|Texas Instruments Incorporated
|tmux7348f,  ±60-V Fault-Protected, 8:1 with configurable fault thresholds
[IBIS Ver]   4.1
[File name]   tmux7348f.ibs
[Date]   01/21/22
[File Rev]   1.0
[Source]
| Texas Instruments Incorporated.
| ASC-INT-MPD
| 12500 TI Blvd
| Dallas, TX - 75243
[Notes]   Revision History:
| Rev 1.0: 01/21/22
| - Initial version of the model
| - Model generated from simulations in SPECTRE
| - C_comp although listed in numerical order of value are
|   obtained from varying PVT conditions. For PVT conditions for
|   each specific value refer the buffer description under
|   respective [Model]. IBIS model user is responsible for using
|   appropriate C_comp to simulate for Signal Integrity.
[Disclaimer]
| This model is designed as an aid for customers of Texas Instruments.
| TI and its licensors and suppliers make no warranties, either expressed
| or implied, with respect to this  model, including the warranties of
| merchantability or fitness for a particular purpose. The model is
| provided solely on an "as is" basis. The entire risk as to its quality
| and performance is with the customer.
| This model is subject to change without notice. Texas Instruments
| Incorporated is not responsible for updating this model.
[Copyright]
(C) Copyright 2022 Texas Instruments Incorporated.All rights reserved.
|  Component TMUX7348FPW 20-pin - PW package
|  Part # TMUX7348FPW
[Component]   TMUX7348FPW
[Manufacturer]  TI
[Package]
|   typ   min   max
R_pkg   0.0668   NA   NA
L_pkg   2.1992nH   NA   NA
C_pkg   0.2884pF   NA   NA
[Pin]   signal_name   model_name
   1   A0   inbuf
   2   EN   inbuf
   3   VSS   POWER
   4   S1   sterm
   5   S2   sterm
   6   S3   sterm
   7   S4   sterm
   8   D   dterm
   9   VFN   nfault
   10   SF   ofault
   11   FF   ofault
   12   VFP   pfault
   13   S8   sterm
   14   S7   sterm
   15   S6   sterm
   16   S5   sterm
   17   VDD   POWER
   18   GND   GND
   19   A2   inbuf
   20   A1   inbuf
[Series Switch Groups]
On 1 /
On 2 /
On 3 /
On 4 /
On 5 /
On 6 /
On 7 /
On 8 /
Off 1 2 3 4 5 6 7 8 /
[Series Pin Mapping]  pin_2 model_name function_table_group
   4   8   switch_dual_20   1
   5   8   switch_dual_20   2
   6   8   switch_dual_20   3
   7   8   switch_dual_20   4
  16   8   switch_dual_20   5
  15   8   switch_dual_20   6
  14   8   switch_dual_20   7
  13   8   switch_dual_20   8
|   4   8   switch_36   1
|   5   8   switch_36   2
|   6   8   switch_36   3
|   7   8   switch_36   4
|  16   8   switch_36   5
|  15   8   switch_36   6
|  14   8   switch_36   7
|  13   8   switch_36   8
|   4   8   switch_dual_15   1
|   5   8   switch_dual_15   2
|   6   8   switch_dual_15   3
|   7   8   switch_dual_15   4
|  16   8   switch_dual_15   5
|  15   8   switch_dual_15   6
|  14   8   switch_dual_15   7
|  13   8   switch_dual_15   8
|   4   8   switch_12   1
|   5   8   switch_12   2
|   6   8   switch_12   3
|   7   8   switch_12   4
|  16   8   switch_12   5
|  15   8   switch_12   6
|  14   8   switch_12   7
|  13   8   switch_12   8
|  Component TMUX7348FRRP 20-pin - RRP package
|  Part # TMUX7348FRRP
[Component]   TMUX7348FRRP
[Manufacturer]  TI
[Package]
|   typ   min   max
R_pkg   0.067   NA   NA
L_pkg   0.937nH   NA   NA
C_pkg   0.144pF   NA   NA
[Pin]   signal_name   model_name
   1   VSS   POWER
   2   S1   sterm
   3   S2   sterm
   4   S3   sterm
   5   S4   sterm
   6   D   dterm
   7   VFN   nfault
   8   SF   ofault
   9   FF   ofault
   10   VFP   pfault
   11   S8   sterm
   12   S7   sterm
   13   S6   sterm
   14   S5   sterm
   15   VDD   POWER
   16   GND   GND
   17   A2   inbuf
   18   A1   inbuf
   19   A0   inbuf
   20   EN   inbuf
[Series Switch Groups]
On 1 /
On 2 /
On 3 /
On 4 /
On 5 /
On 6 /
On 7 /
On 8 /
Off 1 2 3 4 5 6 7 8 /
[Series Pin Mapping]  pin_2 model_name function_table_group
   2   6   switch_dual_20   1
   3   6   switch_dual_20   2
   4   6   switch_dual_20   3
   5   6   switch_dual_20   4
  14   6   switch_dual_20   5
  13   6   switch_dual_20   6
  12   6   switch_dual_20   7
  11   6   switch_dual_20   8
|   2   6   switch_36   1
|   3   6   switch_36   2
|   4   6   switch_36   3
|   5   6   switch_36   4
|  14   6   switch_36   5
|  13   6   switch_36   6
|  12   6   switch_36   7
|  11   6   switch_36   8
|   2   6   switch_dual_15   1
|   3   6   switch_dual_15   2
|   4   6   switch_dual_15   3
|   5   6   switch_dual_15   4
|  14   6   switch_dual_15   5
|  13   6   switch_dual_15   6
|  12   6   switch_dual_15   7
|  11   6   switch_dual_15   8
|   2   6   switch_12   1
|   3   6   switch_12   2
|   4   6   switch_12   3
|   5   6   switch_12   4
|  14   6   switch_12   5
|  13   6   switch_12   6
|  12   6   switch_12   7
|  11   6   switch_12   8
[Model Selector] dterm
dterm_dual_20 Use for operation at +/-20V
dterm_36 Use for operation at 36V
dterm_dual_15 Use for operation at +/-15V
dterm_12 Use for operation at 12V
[Model Selector] ofault
ofault_dual_20 Use for operation at +/-20V
ofault_36 Use for operation at 36V
ofault_dual_15 Use for operation at +/-15V
ofault_12 Use for operation at 12V
[Model Selector] sterm
sterm_dual_20 Use for operation at +/-20V
sterm_36 Use for operation at 36V
sterm_dual_15 Use for operation at +/-15V
sterm_12 Use for operation at 12V
[Model Selector] pfault
pfault_dual_20 Use for operation at +/-20V
pfault_36 Use for operation at 36V
pfault_dual_15 Use for operation at +/-15V
pfault_12 Use for operation at 12V
[Model Selector] inbuf
inbuf_dual_20 Use for operation at +/-20V
inbuf_36 Use for operation at 36V
inbuf_dual_15 Use for operation at +/-15V
inbuf_12 Use for operation at 12V
[Model Selector] nfault
nfault_dual_20 Use for operation at +/-20V
nfault_36 Use for operation at 36V
nfault_dual_15 Use for operation at +/-15V
nfault_12 Use for operation at 12V
| switch_dual_20
[Model]   switch_dual_20
Model_type   Series_switch
|   typ   min   max
C_comp   1.598234e-12   NA   NA
[Voltage Range]   20   NA   NA
[Power Clamp Reference]   20   NA   NA
[Temperature Range]   27   NA   NA
[On]
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[Off]
|   typ   min   max
[R Series]   10G   NA   NA
| switch_36
[Model]   switch_36
Model_type   Series_switch
|   typ   min   max
C_comp   1.598234e-12   NA   NA
[Voltage Range]   36   NA   NA
[Power Clamp Reference]   36   NA   NA
[Temperature Range]   27   NA   NA
[On]
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[Off]
|   typ   min   max
[R Series]   10G   NA   NA
| switch_dual_15
[Model]   switch_dual_15
Model_type   Series_switch
|   typ   min   max
C_comp   1.598234e-12   NA   NA
[Voltage Range]   15   NA   NA
[Power Clamp Reference]   15   NA   NA
[Temperature Range]   27   NA   NA
[On]
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[Off]
|   typ   min   max
[R Series]   10G   NA   NA
| switch_12
[Model]   switch_12
Model_type   Series_switch
|   typ   min   max
C_comp   2.533030e-12   NA   NA
[Voltage Range]   12   NA   NA
[Power Clamp Reference]   12   NA   NA
[Temperature Range]   27   NA   NA
[On]
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[Off]
|   typ   min   max
[R Series]   10G   NA   NA
| Models and submodels in the file (28): ofault_dual_20 (Input), ofault_36 (Input), ofault_dual_15 (Input), ofault_12 (Input), dterm_dual_20 (Terminator), dterm_36 (Terminator), dterm_dual_15 (Terminator), dterm_12 (Terminator), switch_dual_20 (Series_switch), switch_36 (Series_switch), switch_dual_15 (Series_switch), switch_12 (Series_switch), sterm_dual_20 (Terminator), sterm_36 (Terminator), sterm_dual_15 (Terminator), sterm_12 (Terminator), pfault_dual_20 (Input), pfault_36 (Input), pfault_dual_15 (Input), pfault_12 (Input), inbuf_dual_20 (Input), inbuf_36 (Input), inbuf_dual_15 (Input), inbuf_12 (Input), nfault_dual_20 (Input), nfault_36 (Input), nfault_dual_15 (Input), nfault_12 (Input)
